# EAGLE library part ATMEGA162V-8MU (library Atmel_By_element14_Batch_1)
Programmable Flash
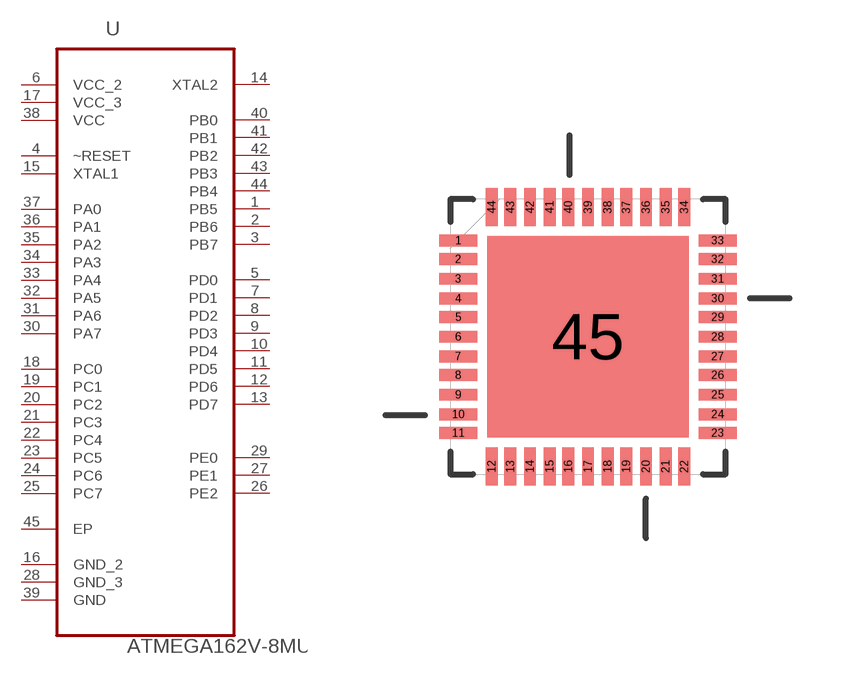
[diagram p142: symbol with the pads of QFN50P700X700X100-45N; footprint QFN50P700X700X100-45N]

Designator prefix U

## ATMEGA162V-8MU (MPN: ATMEGA162V-8MU; OC_FARNELL: 1748512; OC_NEWARK: 26R5625; PACKAGE: QFN-44; SUPPLIER: Atmel)  [QFN50P700X700X100-45N]
1  PB5
2  PB6
3  PB7
4  ~RESET  in
5  PD0
6  VCC_2  pwr
7  PD1
8  PD2
9  PD3
10  PD4
11  PD5
12  PD6
13  PD7
14  XTAL2  out
15  XTAL1  in
16  GND_2  pas
17  VCC_3  pwr
18  PC0
19  PC1
20  PC2
21  PC3
22  PC4
23  PC5
24  PC6
25  PC7
26  PE2
27  PE1
28  GND_3  pas
29  PE0
30  PA7
31  PA6
32  PA5
33  PA4
34  PA3
35  PA2
36  PA1
37  PA0
38  VCC  pwr
39  GND  pas
40  PB0
41  PB1
42  PB2
43  PB3
44  PB4
45  EP  pas

## Footprint QFN50P700X700X100-45N (pad centres in mm)
smd 0.991 x 0.305: 1 -3.353,2.489; 2 -3.353,2.007; 3 -3.353,1.499; 4 -3.353,0.991; 5 -3.353,0.508; 6 -3.353,0; 7 -3.353,-0.508; 8 -3.353,-0.991; 9 -3.353,-1.499; 10 -3.353,-2.007; 11 -3.353,-2.489; 23 3.353,-2.489; 24 3.353,-2.007; 25 3.353,-1.499; 26 3.353,-0.991; 27 3.353,-0.508; 28 3.353,0; 29 3.353,0.508; 30 3.353,0.991; 31 3.353,1.499; 32 3.353,2.007; 33 3.353,2.489
smd 0.305 x 0.991: 12 -2.489,-3.353; 13 -2.007,-3.353; 14 -1.499,-3.353; 15 -0.991,-3.353; 16 -0.508,-3.353; 17 0,-3.353; 18 0.508,-3.353; 19 0.991,-3.353; 20 1.499,-3.353; 21 2.007,-3.353; 22 2.489,-3.353; 34 2.489,3.353; 35 2.007,3.353; 36 1.499,3.353; 37 0.991,3.353; 38 0.508,3.353; 39 0,3.353; 40 -0.508,3.353; 41 -0.991,3.353; 42 -1.499,3.353; 43 -2.007,3.353; 44 -2.489,3.353
smd 5.207 x 5.207: 45 0,0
